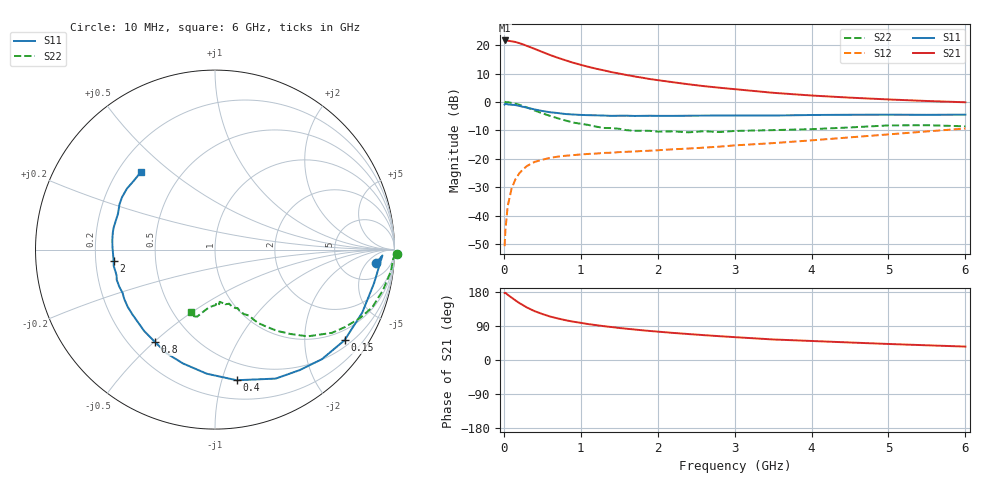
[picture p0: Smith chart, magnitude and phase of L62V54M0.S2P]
!  INFINEON TECHNOLOGIES Small Signal Semiconductors
! BFR380L3 , Si-NPN RF-Transistor in TSLP-3-1
!  Vce=2.5 V,  Ic=4 mA
! Common Emitter S-Parameters:  07. March 2005
#  GHz  S  MA  R  50
! f  S11  S21  S12  S22
! GHz  Mag  Ang  Mag  Ang  Mag  Ang  Mag  Ang
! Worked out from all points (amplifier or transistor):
!   36 points, 10 MHz to 6 GHz, reference 50 ohm
!   highest |S21| = 21.6 dB at 10 MHz (marker M1)
!   |S21| within 3 dB of that: start of sweep to 404.2 MHz
!   unconditionally stable (mu >= 1): 2.477 GHz to 4.697 GHz
!   at 250 MHz: K = 0.15, MSG = 22.0 dB, |S12| = -23.7 dB
!   at 1.4 GHz: K = 0.71, MSG = 14.2 dB, |S12| = -17.9 dB
!   at 6 GHz: K = 0.93, MSG = 4.6 dB, |S12| = -9.4 dB
!   S11 on the Smith chart (normalised r, x): 10 MHz: 12, -9; 150 MHz: 0.67, -3.04; 400 MHz: 0.35, -1.12; 800 MHz: 0.30, -0.50; 2 GHz: 0.28, -0.05; 6 GHz: 0.29, +0.40
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0.01  0.8997 -4.8  12.07 176.8  0.0029 90.0  1.013 -1.4
0.02  0.9333 -2.0  12.03 177.3  0.0055 93.1  0.9937 -2.9
0.05  0.9056 -12.0  11.96 172.2  0.0147 86.1  0.9881 -6.9
0.1  0.8923 -23.2  11.67 164.8  0.0297 78.3  0.9632 -13.5
0.15  0.8808 -35.0  11.35 157.5  0.0434 71.9  0.9338 -20.1
0.2  0.853 -45.7  10.84 150.5  0.0553 67.1  0.8926 -25.4
0.25  0.8206 -54.9  10.29 144.6  0.0652 61.8  0.843 -30.8
0.3  0.7943 -64.8  9.681 138.6  0.0746 58.1  0.8002 -35.4
0.4  0.7377 -80.6  8.589 128.9  0.0881 51.6  0.7074 -43.1
0.5  0.693 -93.8  7.577 121.4  0.0961 47.1  0.6306 -48.2
0.6  0.659 -105.7  6.697 114.8  0.1038 43.6  0.5687 -52.7
0.8  0.6133 -123.2  5.409 105.1  0.113 39.8  0.4727 -59.7
0.9  0.6012 -131.0  4.902 101.2  0.1159 38.8  0.4336 -61.7
1.1  0.5851 -141.8  4.144 94.7  0.1217 38.3  0.3934 -65.9
1.5  0.5719 -158.9  3.154 84.5  0.1309 39.4  0.3369 -72.6
2  0.5685 -173.6  2.419 74.9  0.141 42.8  0.3002 -80.6
2.2  0.5686 -177.8  2.22 71.5  0.1468 44.4  0.3035 -80.9
2.8  0.5772 170.4  1.78 62.9  0.1634 49.9  0.2953 -88.7
3.5  0.5764 159.6  1.448 54.2  0.1886 54.1  0.3193 -94.5
4.5  0.5947 150.5  1.19 46.2  0.2381 59.9  0.3559 -101.2
5.5  0.5931 139.8  1.039 38.8  0.3029 61.4  0.3896 -107.6
6  0.5978 133.6  0.986 35.4  0.3405 60.7  0.3723 -111.0
